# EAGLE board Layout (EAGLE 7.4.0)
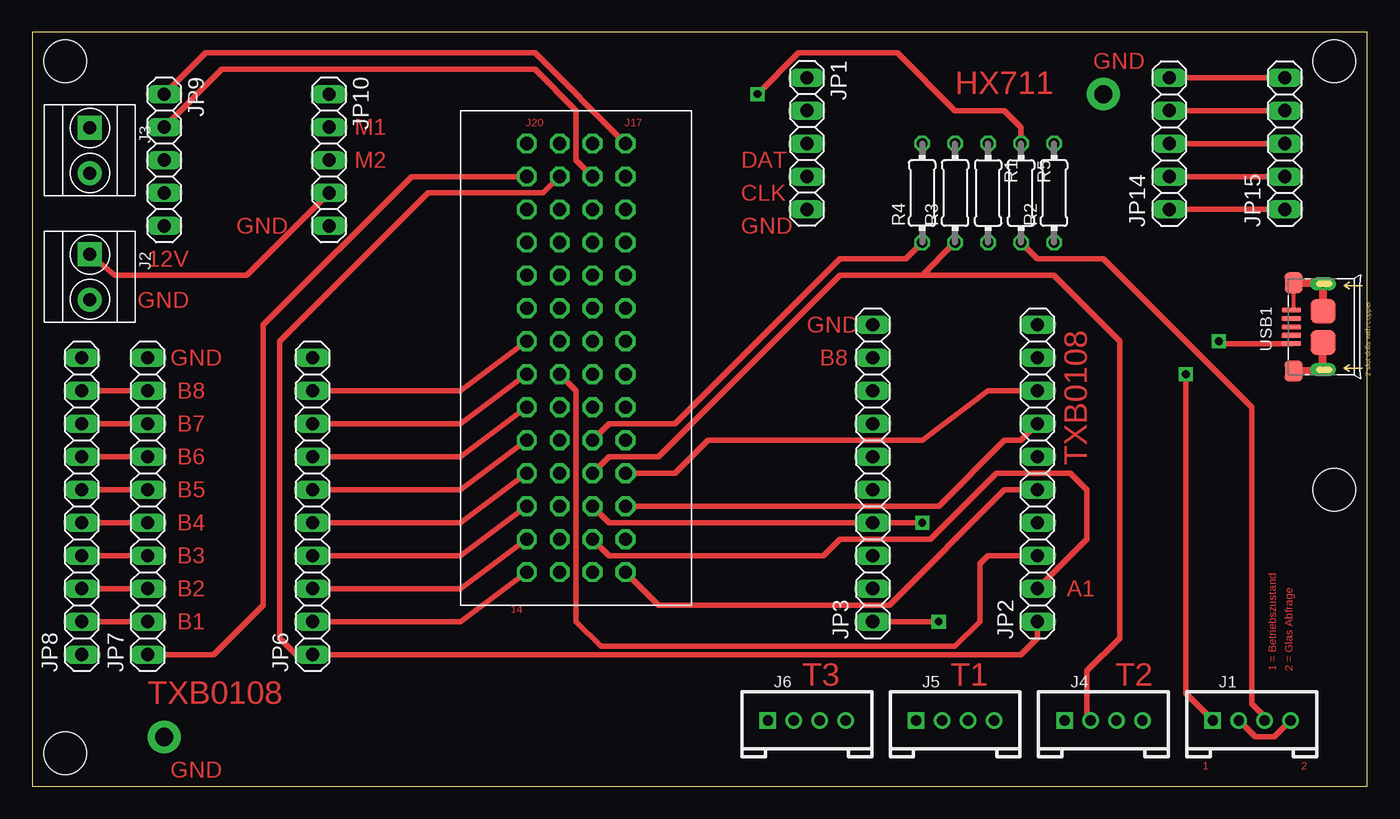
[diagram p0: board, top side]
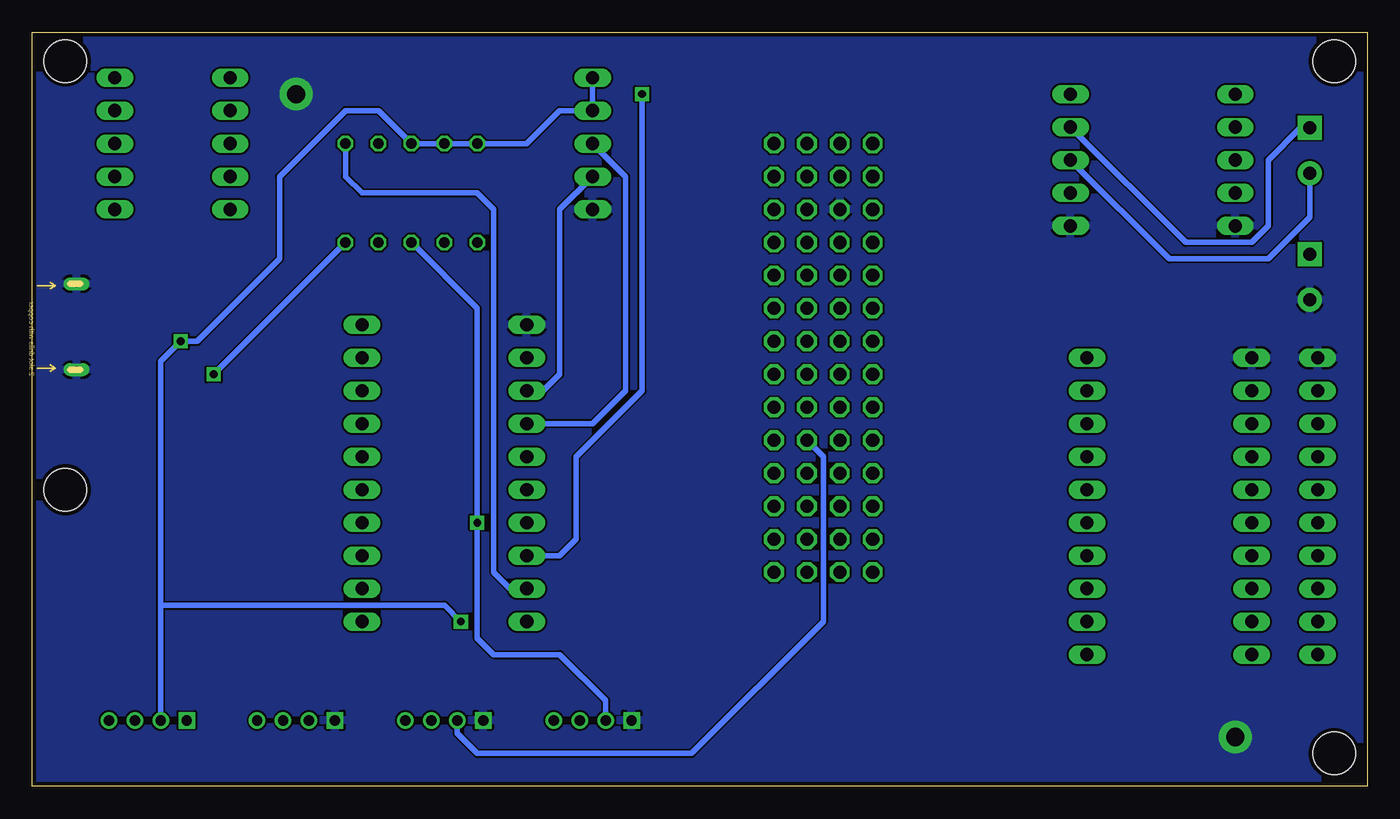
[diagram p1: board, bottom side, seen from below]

Size 102.87 x 58.09 mm. Coordinates in mm from the lower left corner, seen from the top.
Outline: 0,0 102.87,0 102.87,58.09 0,58.09 0,0
Copper layers (1*16): Top 0.035mm / dielectric 1.5mm / Bottom 0.035mm
Design rules "PCB-POOL Standard": minimum track width 0.15mm, minimum drill 0.3mm, track to track 0.15mm, track to pad 0.15mm, pad to pad 0.15mm, via to via 0.15mm, smd to smd 0.15mm, copper to edge 0.3mm, drill to drill 0.2mm, minimum pad ring 0.2mm, minimum via ring 0.15mm, stop-mask expansion 0.075mm, vias tented up to drill 0mil, thermal gap 0.2mm
Holes 3.3 mm at 2.54,55.88 2.54,2.54 100.33,22.86 100.33,55.88

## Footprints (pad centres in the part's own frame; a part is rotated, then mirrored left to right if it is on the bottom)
EDSION_PACKAGE = drill 1.016 pad 1.524 octagon: P$1 17.78,-2.54; P$2 15.24,-2.54; P$3 12.7,-2.54; P$4 10.16,-2.54; P$5 7.62,-2.54; P$6 5.08,-2.54; P$7 2.54,-2.54; P$8 0,-2.54; P$9 -2.54,-2.54; P$10 -5.08,-2.54; P$11 -7.62,-2.54; P$12 -10.16,-2.54; P$13 -12.7,-2.54; P$14 -15.24,-2.54; P$15 17.78,0; P$16 15.24,0; P$17 12.7,0; P$18 10.16,0; P$19 7.62,0; P$20 5.08,0; P$21 2.54,0; P$22 0,0; P$23 -2.54,0; P$24 -5.08,0; P$25 -7.62,0; P$26 -10.16,0; P$27 -12.7,0; P$28 -15.24,0; P$29 17.78,2.54; P$30 15.24,2.54; P$31 12.7,2.54; P$32 10.16,2.54; P$33 7.62,2.54; P$34 5.08,2.54; P$35 2.54,2.54; P$36 0,2.54; P$37 -2.54,2.54; P$38 -5.08,2.54; P$39 -7.62,2.54; P$40 -10.16,2.54; P$41 -12.7,2.54; P$42 -15.24,2.54; P$43 17.78,5.08; P$44 15.24,5.08; P$45 12.7,5.08; P$46 10.16,5.08; P$47 7.62,5.08; P$48 5.08,5.08; P$49 2.54,5.08; P$50 0,5.08; P$51 -2.54,5.08; P$52 -5.08,5.08; P$53 -7.62,5.08; P$54 -10.16,5.08; P$55 -12.7,5.08; P$56 -15.24,5.08
HW4-2.0 = drill 0.8 pad 1.27 square: 1 -3,0 | drill 0.8 pad 1.27: 2 -1,0; 3 1,0; 4 3,0
H2-3.5-7.0X7.0MM = drill 1 pad 1.85 square: 1 -1.75,0 | drill 1 pad 1.85: 2 1.75,0
1X05 = drill 1.016 long: 1 -5.08,0; 2 -2.54,0; 3 0,0; 4 2.54,0; 5 5.08,0
1X10 = drill 1.016 long: 1 -11.43,0; 2 -8.89,0; 3 -6.35,0; 4 -3.81,0; 5 -1.27,0; 6 1.27,0; 7 3.81,0; 8 6.35,0; 9 8.89,0; 10 11.43,0
0204/7 = drill 0.813 octagon: 1 -3.81,0; 2 3.81,0
MICRO-USB5+6P-SMD-0.65-B = smd 0.4 x 1.5: 1 -1.3,-0.25; 2 -0.65,-0.25; 3 0,-0.25; 4 0.65,-0.25; 5 1.3,-0.25 | smd 1.6 x 1.4: S1 -3.4,-0.427; S6 3.4,-0.427 | drill 0.508 pad 1.016 long: S2 -3.3,-2.675; S5 3.3,-2.675 | smd 1.9 x 1.9: S3 -1.2,-2.675; S4 1.2,-2.675

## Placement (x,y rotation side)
IC1  EDISON  [EDSION_PACKAGE]  40.64,34.29 270 top
J1  4P-2.0  [HW4-2.0]  93.98,5.08 0 top
J2  GREEN-2P-3.5  [H2-3.5-7.0X7.0MM]  4.42,39.26 270 top
J3  GREEN-2P-3.5  [H2-3.5-7.0X7.0MM]  4.42,49 270 top
J4  4P-2.0  [HW4-2.0]  82.55,5.08 0 top
J5  4P-2.0  [HW4-2.0]  71.12,5.08 0 top
J6  4P-2.0  [HW4-2.0]  59.69,5.08 0 top
JP1  [1X05]  59.69,49.53 270 top
JP2  [1X10]  77.47,24.13 90 top
JP3  [1X10]  64.77,24.13 90 top
JP6  [1X10]  21.59,21.59 90 top
JP7  [1X10]  8.89,21.59 90 top
JP8  [1X10]  3.81,21.59 90 top
JP9  [1X05]  10.16,48.26 270 top
JP10  [1X05]  22.86,48.26 270 top
JP14  [1X05]  87.63,49.53 90 top
JP15  [1X05]  96.52,49.53 90 top
R1  3k3  [0204/7]  73.66,45.72 270 top
R2  110  [0204/7]  78.74,45.72 90 top
R3  3k3  [0204/7]  71.12,45.72 90 top
R4  3k3  [0204/7]  68.58,45.72 90 top
R5  110  [0204/7]  76.2,45.72 270 top
USB1  10118193-0001LF  [MICRO-USB5+6P-SMD-0.65-B]  96.79,35.41 90 top

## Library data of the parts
IC1 = edison
J1-J6 = Seeed-Connector -2016
JP1-JP3 JP6-JP10 JP14 JP15 = pinhead
R1-R5 = rcl
USB1 = Seeed-Connector -2016; MPN: 10118193-0001LF

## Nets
+3V3: IC1.P$13 JP7.1
+5V: J1.2 J1.4 JP1.1 JP1.2 JP3.1 R1.1 R3.2 R4.2 USB1.1
+12V: J2.1 JP10.4
BLK: JP14.2 JP15.2
DIR: IC1.P$41 JP9.2
GND: IC1.P$26 J2.2 J4.1 J5.1 J6.1 JP1.5 JP3.10 JP7.10 JP8.10 JP9.5 JP10.5 USB1.5 USB1.S1 USB1.S2 USB1.S3 USB1.S4 USB1.S5 USB1.S6
GRN: JP14.4 JP15.4
LOAD_CELL_CLK: JP1.4 JP3.8
LOAD_CELL_CLK_EDI: IC1.P$46 JP2.8
LOAD_CELL_DATA: JP1.3 JP3.7
LOAD_CELL_DATA_EDI: IC1.P$45 JP2.7
M1: J3.1 JP10.2
M2: J3.2 JP10.3
N$1: J1.1 R2.1
N$2: J1.3 R5.2
N$3: JP3.3 R5.1
PWM: IC1.P$56 JP9.1
RED: JP14.1 JP15.1
TASTER_1: IC1.P$33 J5.2 R4.1
TASTER_2: IC1.P$32 J4.2 R3.1
TASTER_3: IC1.P$31 J6.2 JP3.4 R1.2
TXB0104_A1: IC1.P$30 JP2.2
TXB0104_A2: IC1.P$21 JP2.3
TXB0104_A4: IC1.P$43 JP2.5
TXB0104_B1: JP3.2 R2.2
TXB0108_A1: IC1.P$1 JP6.2
TXB0108_A2: IC1.P$2 JP6.3
TXB0108_A3: IC1.P$3 JP6.4
TXB0108_A4: IC1.P$4 JP6.5
TXB0108_A5: IC1.P$5 JP6.6
TXB0108_A6: IC1.P$6 JP6.7
TXB0108_A7: IC1.P$7 JP6.8
TXB0108_A8: IC1.P$8 JP6.9
TXB0108_B1: JP7.2 JP8.2
TXB0108_B2: JP7.3 JP8.3
TXB0108_B3: JP7.4 JP8.4
TXB0108_B4: JP7.5 JP8.5
TXB0108_B5: JP7.6 JP8.6
TXB0108_B6: JP7.7 JP8.7
TXB0108_B7: JP7.8 JP8.8
TXB0108_B8: JP7.9 JP8.9
VDD: IC1.P$27 JP2.1 JP6.1
WHT: JP14.3 JP15.3
YLW: JP14.5 JP15.5

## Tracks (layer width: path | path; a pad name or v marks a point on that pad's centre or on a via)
+3V3
  Top 0.406: IC1.P$13 29.21,46.99 17.78,35.56 17.78,13.97 13.97,10.16 JP7.1
+5V  (via drill 0.6)
  Top 0.406: J1.2 94.25,3.81 95.71,3.81 J1.4 | USB1.1 91.62,34.11 v91.44,34.29 | v69.85,12.7 JP3.1
  Bottom 0.406: JP1.1 JP1.2 62.23,52.07 64.77,49.53 R4.2 R3.2 R1.1 76.2,52.07 78.74,52.07 83.82,46.99 83.82,40.64 90.17,34.29 v91.44,34.29 | 92.98,13.97 71.12,13.97 v69.85,12.7 | 91.71,34.02 v91.44,34.29 | J1.2 92.98,13.97 | 92.98,13.97 92.98,32.75 v91.44,34.29
+12V
  Top 0.406: J2.1 6.35,39.37 16.51,39.37 JP10.4
BLK
  Top 0.406: JP14.2 JP15.2
DIR
  Top 0.406: IC1.P$41 41.91,48.26 41.91,52.07 38.73,55.24 14.61,55.24 JP9.2
GND  (via drill 1.4)
  Top 0.3: 99.37,36.71 USB1.S4 | USB1.5 97.22,36.89 USB1.S6
  Top 0.6: USB1.S6 99.37,38.81 USB1.S5 USB1.S4 | USB1.S3 USB1.S2 99.37,32.01 USB1.S1
  other vias: 10.16,3.81 82.55,53.34
  pour Bottom: -1.07,58.15 105.41,58.15 105.41,-1.27 -1.07,-1.27
GRN
  Top 0.406: JP14.4 JP15.4
LOAD_CELL_CLK
  Bottom 0.406: JP1.4 62.23,44.45 62.23,31.75 63.5,30.48 JP3.8
LOAD_CELL_CLK_EDI
  Top 0.406: IC1.P$46 49.53,24.13 52.07,26.67 68.58,26.67 73.66,30.48 JP2.8
LOAD_CELL_DATA
  Bottom 0.406: JP1.3 57.15,46.99 57.15,30.48 59.69,27.94 JP3.7
LOAD_CELL_DATA_EDI
  Top 0.406: IC1.P$45 69.85,21.59 74.93,26.67 76.2,26.67 JP2.7
M1
  Bottom 0.406: J3.1 5.13,50.75 7.62,48.26 7.62,43.18 8.89,41.91 13.97,41.91 JP10.2
M2
  Bottom 0.406: J3.2 4.42,43.84 7.62,40.64 15.24,40.64 JP10.3
N$1  (via drill 0.6)
  Top 0.406: v88.9,31.75 88.9,7.16 J1.1
  Bottom 0.406: R2.1 v88.9,31.75
N$2
  Top 0.406: R5.2 77.47,40.64 82.55,40.64 93.98,29.21 93.98,6.35 95.25,5.08 J1.3
N$3  (via drill 0.6)
  Top 0.406: R5.1 76.2,50.8 74.93,52.07 71.12,52.07 66.67,56.52 59.05,56.52 v55.88,53.34
  Bottom 0.406: JP3.3 62.23,17.78 60.96,19.05 60.96,25.4 55.88,30.48 v55.88,53.34
PWM
  Top 0.406: IC1.P$56 38.73,56.52 13.34,56.52 JP9.1
RED
  Top 0.406: JP14.1 JP15.1
TASTER_1
  Top 0.406: R4.1 67.31,40.64 62.23,40.64 49.53,27.94 44.45,27.94 IC1.P$33
  Bottom 0.406: IC1.P$33 41.91,25.4 41.91,12.7 52.07,2.54 68.58,2.54 70.12,4.08 J5.2
TASTER_2
  Top 0.406: R3.1 68.58,39.37 | 68.58,39.37 62.23,39.37 48.26,25.4 44.45,25.4 IC1.P$32 | 68.58,39.37 78.74,39.37 83.82,34.29 83.82,11.43 81.28,8.89 81.28,5.35 J4.2
TASTER_3  (via drill 0.6)
  Top 0.406: v68.58,20.32 JP3.4 44.45,20.32 IC1.P$31
  Bottom 0.406: R1.2 68.58,36.83 v68.58,20.32 68.58,11.43 67.31,10.16 62.23,10.16 58.69,6.62 J6.2
TXB0104_A1
  Top 0.406: JP2.2 81.28,19.05 81.28,22.86 80.01,24.13 74.3,24.13 69.22,19.05 62.23,19.05 60.96,17.78 44.45,17.78 IC1.P$30
TXB0104_A2
  Top 0.406: JP2.3 73.66,17.78 73.03,17.14 73.03,12.7 71.12,10.79 43.81,10.79 41.91,12.7 41.91,30.48 IC1.P$21
TXB0104_A4
  Top 0.406: JP2.5 74.93,22.86 66.04,13.97 48.26,13.97 IC1.P$43
TXB0104_B1
  Bottom 0.406: R2.2 78.74,46.99 77.47,45.72 68.58,45.72 67.31,44.45 67.31,16.51 66.04,15.24 JP3.2
TXB0108_A1
  Top 0.406: JP6.2 33.02,12.7 IC1.P$1
TXB0108_A2
  Top 0.406: JP6.3 33.02,15.24 IC1.P$2
TXB0108_A3
  Top 0.406: JP6.4 33.02,17.78 IC1.P$3
TXB0108_A4
  Top 0.406: JP6.5 33.02,20.32 IC1.P$4
TXB0108_A5
  Top 0.406: JP6.6 33.02,22.86 IC1.P$5
TXB0108_A6
  Top 0.406: JP6.7 33.02,25.4 IC1.P$6
TXB0108_A7
  Top 0.406: JP6.8 33.02,27.94 IC1.P$7
TXB0108_A8
  Top 0.406: JP6.9 33.02,30.48 IC1.P$8
TXB0108_B1
  Top 0.406: JP8.2 JP7.2
TXB0108_B2
  Top 0.406: JP8.3 JP7.3
TXB0108_B3
  Top 0.406: JP8.4 JP7.4
TXB0108_B4
  Top 0.406: JP8.5 JP7.5
TXB0108_B5
  Top 0.406: JP8.6 JP7.6
TXB0108_B6
  Top 0.406: JP8.7 JP7.7
TXB0108_B7
  Top 0.406: JP8.8 JP7.8
TXB0108_B8
  Top 0.406: JP8.9 JP7.9
VDD
  Top 0.406: JP2.1 77.47,11.43 76.2,10.16 JP6.1 20.32,10.16 19.05,11.43 19.05,34.29 30.48,45.72 39.37,45.72 IC1.P$27
WHT
  Top 0.406: JP14.3 JP15.3
YLW
  Top 0.406: JP14.5 JP15.5

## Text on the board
Top: GND | HX711 | M1 | J20 | J17 | M2 | DAT | CLK | GND | GND | 12V | GND | GND | GND | B8 | B8 | B7 | B6 | TXB0108 | B5 | B4 | B3 | B2 | A1 | B1 | 14 | T3 | T1 | T2 | 1 = Betriebszustand | 2 = Glas Abfrage | TXB0108 | GND | 1 | 2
